(* Logix 5000 AddOnInstructionDefinition export HI6500_Faceplate_AOI; software revision 28.00 *)

ADD_ON_INSTRUCTION HI6500_Faceplate_AOI   (* revision 1.2 *)
VAR_IN_OUT
   Inp_hi6500 : _0102:Hardy6500Series_19FEEB66:I:0; {required}
   Out_hi6500 : _0102:Hardy6500Series_74A2D67F:O:0; {required}
END_VAR
VAR_OUTPUT
   hardy_6500_net_wt : REAL; {access Read Only}
   hardy_6500_counter : SINT; {access Read Only}
   hardy_6500_gross_wt : REAL; {access Read Only}
   hardy_6500_status : DINT; {access Read Only}
   hardy_6500_unit_status : INT; {access Read Only}
END_VAR
VAR_INPUT
   Set_FaceplateAnimation : DINT;
   rd_c2_cal : DINT;
   pm_4081 : DINT;
   pm_4082 : REAL;
   pm_4103 : DINT;
   pm_4101 : REAL;
   pm_4102 : REAL;
   rd_tra_cal : DINT;
   pm_4181 : REAL;
   pm_4182 : REAL;
   rd_fill : DINT;
   pm_2081 : DINT;
   pm_2082 : DINT;
   rd_ins : DINT;
   pm_2882 : DINT;
   pm_2883 : DINT;
   pm_2887 : REAL;
   pm_2888 : REAL;
   pm_2881 : DINT;
   rd_op2 : DINT;
   pm_2886 : REAL;
   pm_6182 : REAL;
   pm_6183 : REAL;
   pm_6303 : REAL;
   rd_az : DINT;
   pm_6301 : DINT;
   pm_6302 : REAL;
   pm_6381 : REAL;
   rd_iz : DINT;
   pm_6281 : DINT;
   pm_6282 : REAL;
   pm_6283 : REAL;
   pm_6284 : REAL;
   zero_cmd1 : DINT;
   tare_cmd : DINT;
   cal_low_cmd : DINT;
   cal_high_cmd : DINT;
   c2_cmd : DINT;
   control_bit : DINT;
   wr_cal_m_tol : DINT;
   fp_dis_md : DINT := 4;
   tare_zero_cmd : DINT;
   tare_zero_vl : DINT;
   wr_cell_sens : DINT;
   wr_wav_sav : DINT;
   wr_num_avg : DINT;
   wr_dec_pt : DINT;
   wr_grad : DINT;
   wr_mot_tol : DINT;
   wr_scal_cap : DINT;
   wr_unit : DINT;
   wr_ct_ena : DINT;
   pm_6104 : DINT;
   wr_un_wt : DINT;
   pm_6102 : REAL;
   wr_sm_size : DINT;
   pm_6103 : DINT;
   wr_dis_md : DINT;
   pm_8083 : DINT;
   wr_zr_tol : DINT;
   wr_tr_off : DINT;
   wr_tr_amt : DINT;
   wr_ref_wt : DINT;
   wr_gra_corr : DINT;
   wr_cal_lo_wt : DINT;
   wr_span_wt : DINT;
   wr_az_enable : DINT;
   wr_az_tol : DINT;
   wr_warm_time : DINT;
   wr_iz_enable : DINT;
   wr_plusiz_tol : DINT;
   wr_minusiz_tol : DINT;
   save_ins_pm : DINT;
   save_c2_pm : INT;
   save_op2_pm : INT;
   save_az_pm : INT;
   save_iz_pm : INT;
   save_tradcal_pm : INT;
   pm_6201 : REAL;
   Set_FaceplateHelpAnimation : DINT;
   wr_cal_m_tol_2 : INT;
   wr_nvm_cmd : DINT;
END_VAR
VAR_OUTPUT
   unit_flt : BOOL; {access Read Only}
   cal_status : DINT := 20; {access Read Only}
   status1 : DINT; {access Read Only}
END_VAR
VAR_INPUT
   save_fil_pm : INT;
END_VAR
VAR_OUTPUT
   instrument_status : DINT; {access Read Only}
END_VAR
VAR
   start_timer4 : BOOL; {access None}
   delay4 : TIMER := (PRE := 200); {access None}
   start_timer2 : BOOL; {access None}
   delay2 : TIMER := (PRE := 200); {access None}
   start_timer5 : BOOL; {access None}
   delay5 : TIMER := (PRE := 200); {access None}
   start_timer : BOOL; {access None}
   delay : TIMER := (PRE := 200); {access None}
   start_timer7 : BOOL; {access None}
   delay7 : TIMER := (PRE := 200); {access None}
   start_timer6 : BOOL; {access None}
   delay6 : TIMER := (PRE := 200); {access None}
   start_timer8 : BOOL; {access None}
   delay8 : TIMER := (PRE := 200); {access None}
   cmd_no : DINT; {access None}
   start_timer9 : BOOL; {access None}
   delay9 : TIMER := (PRE := 200); {access None}
   start_timer10 : BOOL; {access None}
   delay10 : TIMER := (PRE := 200); {access None}
   start_timer11 : BOOL; {access None}
   delay11 : TIMER := (PRE := 200); {access None}
   start_timer12 : BOOL; {access None}
   delay12 : TIMER := (PRE := 200); {access None}
   start_timer13 : BOOL; {access None}
   delay13 : TIMER := (PRE := 200); {access None}
   start_timer14 : BOOL; {access None}
   delay14 : TIMER := (PRE := 200); {access None}
   start_timer15 : BOOL; {access None}
   delay15 : TIMER := (PRE := 200); {access None}
   start_timer16 : BOOL; {access None}
   delay16 : TIMER := (PRE := 200); {access None}
   start_timer17 : BOOL; {access None}
   delay17 : TIMER := (PRE := 200); {access None}
   start_timer18 : BOOL; {access None}
   delay18 : TIMER := (PRE := 200); {access None}
   start_timer19 : BOOL; {access None}
   delay19 : TIMER := (PRE := 200); {access None}
   start_timer20 : BOOL; {access None}
   delay20 : TIMER := (PRE := 200); {access None}
   start_timer21 : BOOL; {access None}
   delay21 : TIMER := (PRE := 200); {access None}
   start_timer22 : BOOL; {access None}
   delay22 : TIMER := (PRE := 200); {access None}
   start_timer23 : BOOL; {access None}
   delay23 : TIMER := (PRE := 200); {access None}
   start_timer24 : BOOL; {access None}
   delay24 : TIMER := (PRE := 200); {access None}
   start_timer25 : BOOL; {access None}
   delay25 : TIMER := (PRE := 80); {access None}
   cmd_no_cal : DINT; {access None}
   start_timer26 : BOOL; {access None}
   delay26 : TIMER := (PRE := 200); {access None}
   start_timer27 : BOOL; {access None}
   delay27 : TIMER := (PRE := 200); {access None}
   start_timer28 : BOOL; {access None}
   delay28 : TIMER := (PRE := 200); {access None}
   start_timer29 : BOOL; {access None}
   delay29 : TIMER := (PRE := 200); {access None}
   start_timer30 : BOOL; {access None}
   delay30 : TIMER := (PRE := 200); {access None}
   wr_cell_sens2 : INT; {access None}
   start_timer31 : BOOL; {access None}
   delay31 : TIMER := (PRE := 200); {access None}
   start_timer32 : BOOL; {access None}
   delay32 : TIMER := (PRE := 200); {access None}
   start_timer33 : BOOL; {access None}
   delay33 : TIMER := (PRE := 200); {access None}
   temp : BOOL; {access None}
   temp3 : BOOL; {access None}
   timer35 : TIMER := (PRE := 4000); {access None}
   temp2 : BOOL; {access None}
   temp4 : BOOL; {access None}
   temp5 : BOOL; {access None}
   temp6 : BOOL; {access None}
   temp7 : BOOL; {access None}
   temp8 : BOOL; {access None}
   temp9 : BOOL; {access None}
   temp10 : BOOL; {access None}
   temp11 : BOOL; {access None}
   temp12 : BOOL; {access None}
   temp13 : BOOL; {access None}
   temp14 : BOOL; {access None}
   temp15 : BOOL; {access None}
   temp16 : BOOL; {access None}
   temp17 : BOOL; {access None}
   temp18 : BOOL; {access None}
   temp19 : BOOL; {access None}
   temp20 : BOOL; {access None}
   temp21 : BOOL; {access None}
   temp22 : BOOL; {access None}
   temp23 : BOOL; {access None}
   temp24 : BOOL; {access None}
   temp25 : BOOL; {access None}
   temp26 : BOOL; {access None}
   temp27 : BOOL; {access None}
   temp28 : BOOL; {access None}
   temp29 : BOOL; {access None}
   temp100 : BOOL; {access None}
   blk : BOOL; {access None}
   timer38 : TIMER := (PRE := 2000); {access None}
   timer39 : TIMER := (PRE := 2000); {access None}
   temp42 : BOOL; {access None}
   temp41 : BOOL; {access None}
END_VAR

ROUTINE Logic   (* ladder *)
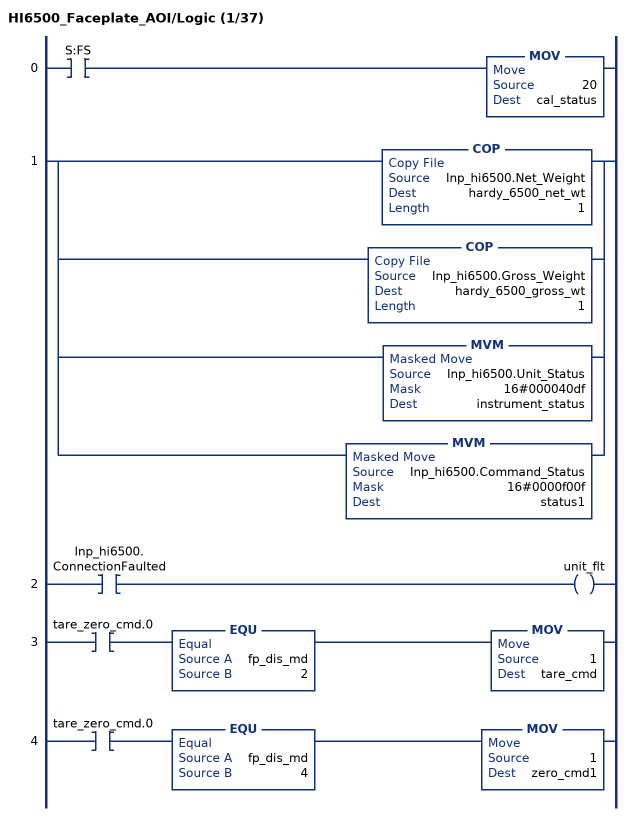
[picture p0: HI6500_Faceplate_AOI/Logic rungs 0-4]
   0: XIC(S:FS)MOV(20,cal_status);
   1: [COP(Inp_hi6500.Net_Weight,hardy_6500_net_wt,1) ,COP(Inp_hi6500.Gross_Weight,hardy_6500_gross_wt,1) ,MVM(Inp_hi6500.Unit_Status,16#000040df,instrument_status) ,MVM(Inp_hi6500.Command_Status,16#0000f00f,status1) ];
   2: XIC(Inp_hi6500.ConnectionFaulted)OTE(unit_flt);
   3: XIC(tare_zero_cmd.0)EQU(fp_dis_md,2)MOV(1,tare_cmd);
   4: XIC(tare_zero_cmd.0)EQU(fp_dis_md,4)MOV(1,zero_cmd1);
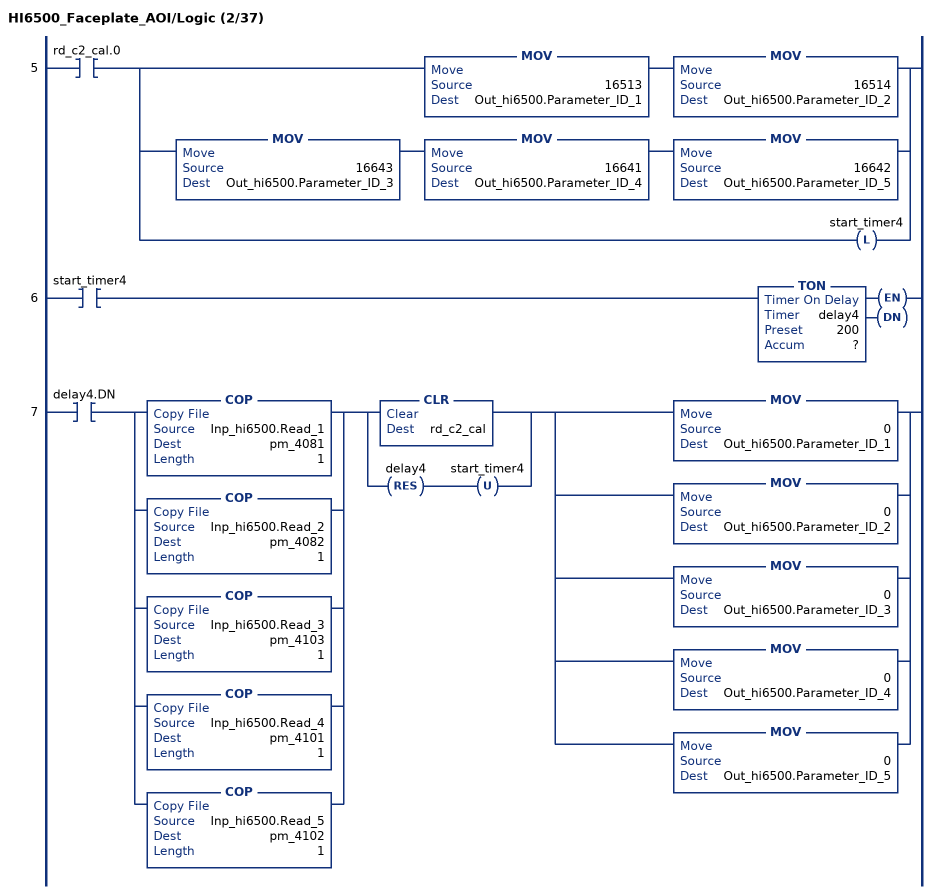
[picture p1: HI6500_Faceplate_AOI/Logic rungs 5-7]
   5: XIC(rd_c2_cal.0)[MOV(16513,Out_hi6500.Parameter_ID_1) MOV(16514,Out_hi6500.Parameter_ID_2) ,MOV(16643,Out_hi6500.Parameter_ID_3) MOV(16641,Out_hi6500.Parameter_ID_4) MOV(16642,Out_hi6500.Parameter_ID_5) ,OTL(start_timer4) ];
   6: XIC(start_timer4)TON(delay4,?,?);
   7: XIC(delay4.DN)[COP(Inp_hi6500.Read_1,pm_4081,1) ,COP(Inp_hi6500.Read_2,pm_4082,1) ,COP(Inp_hi6500.Read_3,pm_4103,1) ,COP(Inp_hi6500.Read_4,pm_4101,1) ,COP(Inp_hi6500.Read_5,pm_4102,1) ][CLR(rd_c2_cal) ,RES(delay4) OTU(start_timer4) ][MOV(0,Out_hi6500.Parameter_ID_1) ,MOV(0,Out_hi6500.Parameter_ID_2) ,MOV(0,Out_hi6500.Parameter_ID_3) ,MOV(0,Out_hi6500.Parameter_ID_4) ,MOV(0,Out_hi6500.Parameter_ID_5) ];
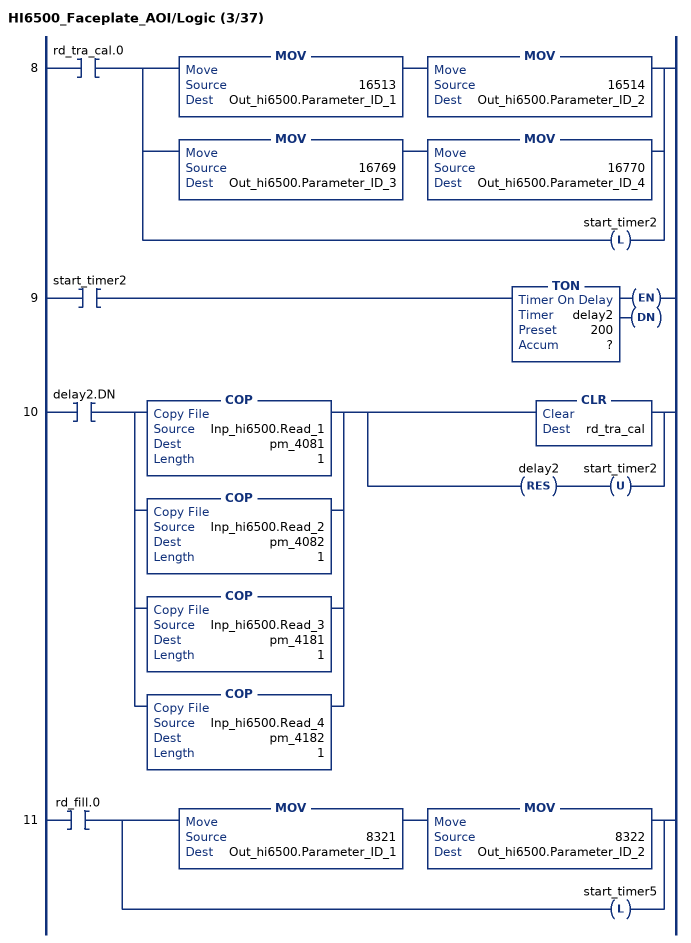
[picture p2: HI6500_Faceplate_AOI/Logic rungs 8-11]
   8: XIC(rd_tra_cal.0)[MOV(16513,Out_hi6500.Parameter_ID_1) MOV(16514,Out_hi6500.Parameter_ID_2) ,MOV(16769,Out_hi6500.Parameter_ID_3) MOV(16770,Out_hi6500.Parameter_ID_4) ,OTL(start_timer2) ];
   9: XIC(start_timer2)TON(delay2,?,?);
   10: XIC(delay2.DN)[COP(Inp_hi6500.Read_1,pm_4081,1) ,COP(Inp_hi6500.Read_2,pm_4082,1) ,COP(Inp_hi6500.Read_3,pm_4181,1) ,COP(Inp_hi6500.Read_4,pm_4182,1) ][CLR(rd_tra_cal) ,RES(delay2) OTU(start_timer2) ];
   11: XIC(rd_fill.0)[MOV(8321,Out_hi6500.Parameter_ID_1) MOV(8322,Out_hi6500.Parameter_ID_2) ,OTL(start_timer5) ];
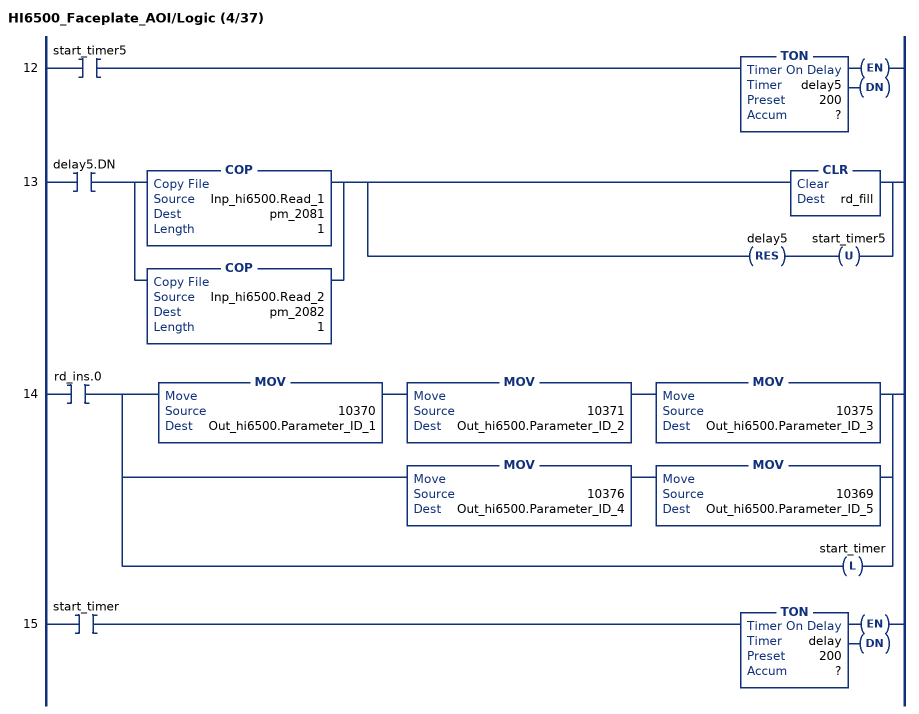
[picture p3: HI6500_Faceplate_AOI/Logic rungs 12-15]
   12: XIC(start_timer5)TON(delay5,?,?);
   13: XIC(delay5.DN)[COP(Inp_hi6500.Read_1,pm_2081,1) ,COP(Inp_hi6500.Read_2,pm_2082,1) ][CLR(rd_fill) ,RES(delay5) OTU(start_timer5) ];
   14: XIC(rd_ins.0)[MOV(10370,Out_hi6500.Parameter_ID_1) MOV(10371,Out_hi6500.Parameter_ID_2) MOV(10375,Out_hi6500.Parameter_ID_3) ,MOV(10376,Out_hi6500.Parameter_ID_4) MOV(10369,Out_hi6500.Parameter_ID_5) ,OTL(start_timer) ];
   15: XIC(start_timer)TON(delay,?,?);
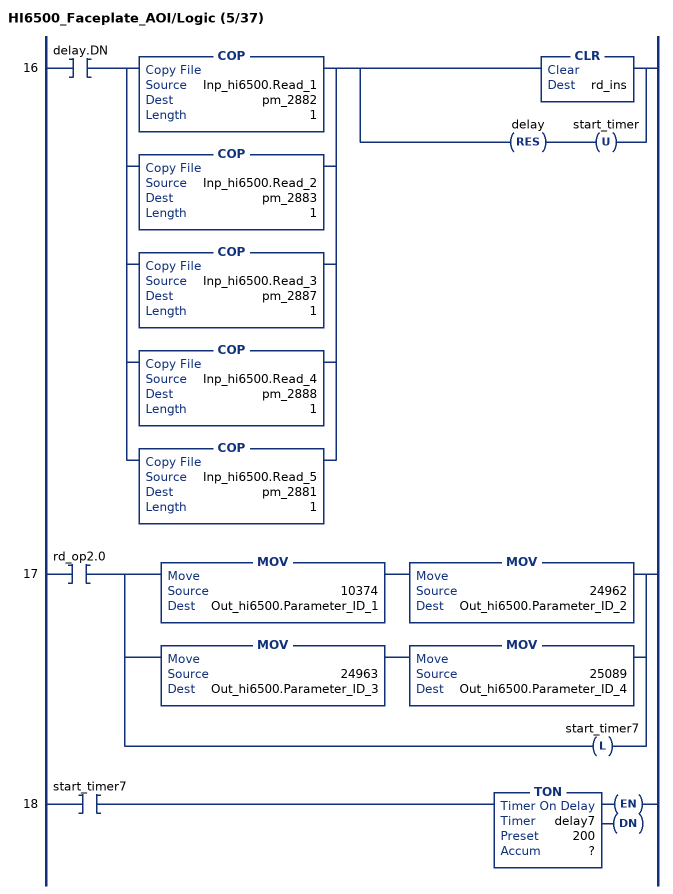
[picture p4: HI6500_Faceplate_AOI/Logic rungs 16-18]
   16: XIC(delay.DN)[COP(Inp_hi6500.Read_1,pm_2882,1) ,COP(Inp_hi6500.Read_2,pm_2883,1) ,COP(Inp_hi6500.Read_3,pm_2887,1) ,COP(Inp_hi6500.Read_4,pm_2888,1) ,COP(Inp_hi6500.Read_5,pm_2881,1) ][CLR(rd_ins) ,RES(delay) OTU(start_timer) ];
   17: XIC(rd_op2.0)[MOV(10374,Out_hi6500.Parameter_ID_1) MOV(24962,Out_hi6500.Parameter_ID_2) ,MOV(24963,Out_hi6500.Parameter_ID_3) MOV(25089,Out_hi6500.Parameter_ID_4) ,OTL(start_timer7) ];
   18: XIC(start_timer7)TON(delay7,?,?);
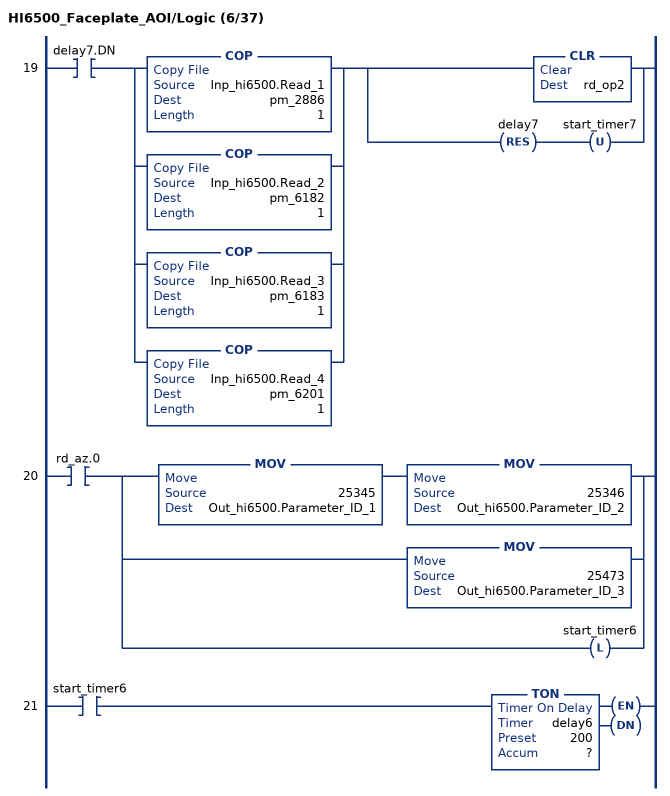
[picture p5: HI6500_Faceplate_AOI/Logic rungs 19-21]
   19: XIC(delay7.DN)[COP(Inp_hi6500.Read_1,pm_2886,1) ,COP(Inp_hi6500.Read_2,pm_6182,1) ,COP(Inp_hi6500.Read_3,pm_6183,1) ,COP(Inp_hi6500.Read_4,pm_6201,1) ][CLR(rd_op2) ,RES(delay7) OTU(start_timer7) ];
   20: XIC(rd_az.0)[MOV(25345,Out_hi6500.Parameter_ID_1) MOV(25346,Out_hi6500.Parameter_ID_2) ,MOV(25473,Out_hi6500.Parameter_ID_3) ,OTL(start_timer6) ];
   21: XIC(start_timer6)TON(delay6,?,?);
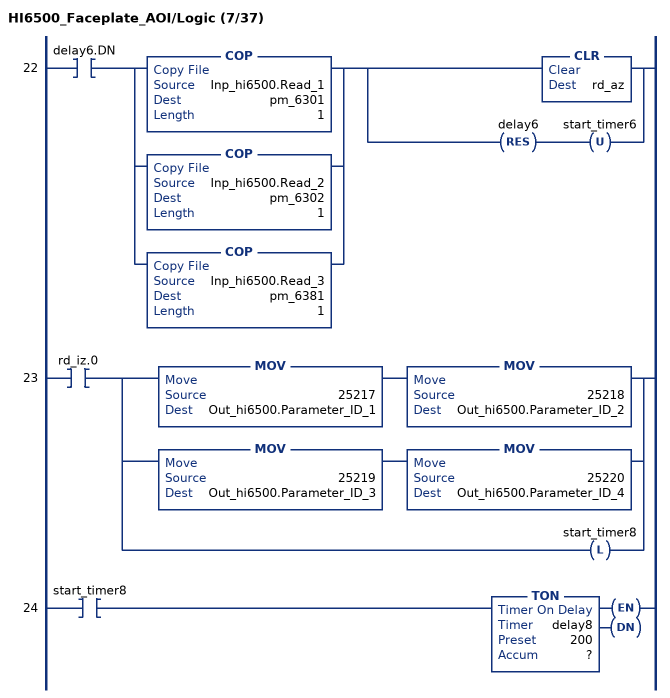
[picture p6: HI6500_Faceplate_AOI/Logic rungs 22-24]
   22: XIC(delay6.DN)[COP(Inp_hi6500.Read_1,pm_6301,1) ,COP(Inp_hi6500.Read_2,pm_6302,1) ,COP(Inp_hi6500.Read_3,pm_6381,1) ][CLR(rd_az) ,RES(delay6) OTU(start_timer6) ];
   23: XIC(rd_iz.0)[MOV(25217,Out_hi6500.Parameter_ID_1) MOV(25218,Out_hi6500.Parameter_ID_2) ,MOV(25219,Out_hi6500.Parameter_ID_3) MOV(25220,Out_hi6500.Parameter_ID_4) ,OTL(start_timer8) ];
   24: XIC(start_timer8)TON(delay8,?,?);
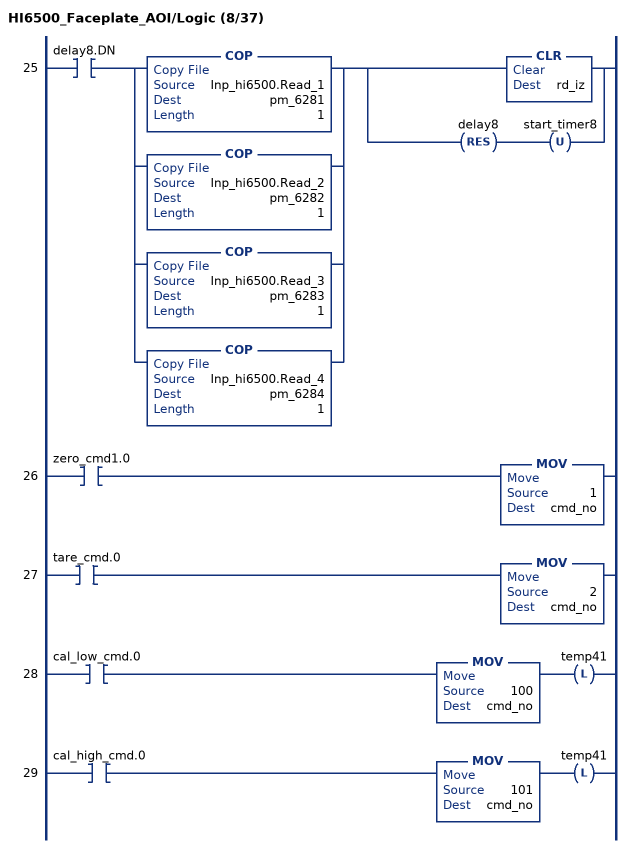
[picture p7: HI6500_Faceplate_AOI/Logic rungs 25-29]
   25: XIC(delay8.DN)[COP(Inp_hi6500.Read_1,pm_6281,1) ,COP(Inp_hi6500.Read_2,pm_6282,1) ,COP(Inp_hi6500.Read_3,pm_6283,1) ,COP(Inp_hi6500.Read_4,pm_6284,1) ][CLR(rd_iz) ,RES(delay8) OTU(start_timer8) ];
   26: XIC(zero_cmd1.0)MOV(1,cmd_no);
   27: XIC(tare_cmd.0)MOV(2,cmd_no);
   28: XIC(cal_low_cmd.0)MOV(100,cmd_no)OTL(temp41);
   29: XIC(cal_high_cmd.0)MOV(101,cmd_no)OTL(temp41);
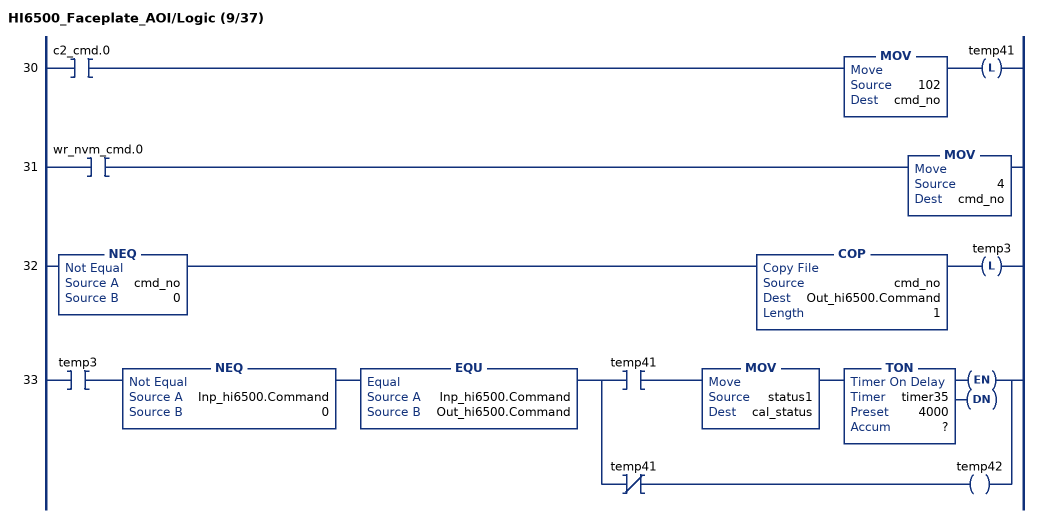
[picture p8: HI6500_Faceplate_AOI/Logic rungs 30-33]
   30: XIC(c2_cmd.0)MOV(102,cmd_no)OTL(temp41);
   31: XIC(wr_nvm_cmd.0)MOV(4,cmd_no);
   32: NEQ(cmd_no,0)COP(cmd_no,Out_hi6500.Command,1)OTL(temp3);
   33: XIC(temp3)NEQ(Inp_hi6500.Command,0)EQU(Inp_hi6500.Command,Out_hi6500.Command)[XIC(temp41) MOV(status1,cal_status) TON(timer35,?,?) ,XIO(temp41) OTE(temp42) ];
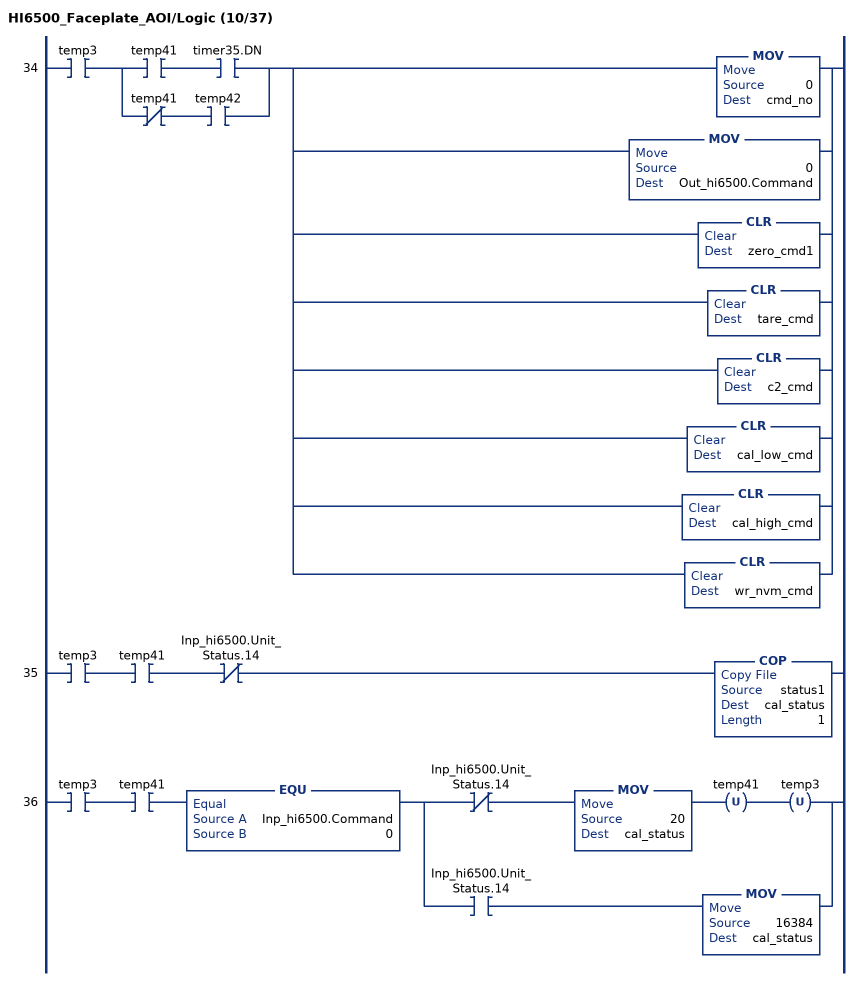
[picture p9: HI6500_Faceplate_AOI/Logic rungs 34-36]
   34: XIC(temp3)[XIC(temp41) XIC(timer35.DN) ,XIO(temp41) XIC(temp42) ][MOV(0,cmd_no) ,MOV(0,Out_hi6500.Command) ,CLR(zero_cmd1) ,CLR(tare_cmd) ,CLR(c2_cmd) ,CLR(cal_low_cmd) ,CLR(cal_high_cmd) ,CLR(wr_nvm_cmd) ];
   35: XIC(temp3)XIC(temp41)XIO(Inp_hi6500.Unit_Status.14)COP(status1,cal_status,1);
   36: XIC(temp3)XIC(temp41)EQU(Inp_hi6500.Command,0)[XIO(Inp_hi6500.Unit_Status.14) MOV(20,cal_status) OTU(temp41) OTU(temp3) ,XIC(Inp_hi6500.Unit_Status.14) MOV(16384,cal_status) ];
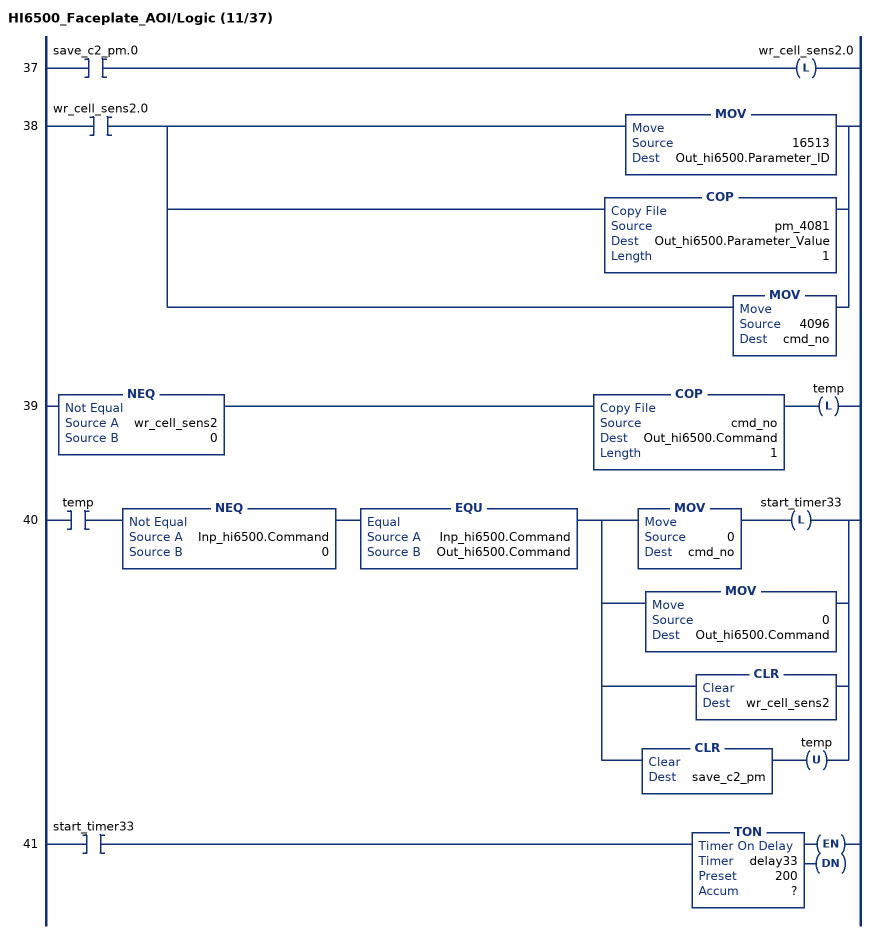
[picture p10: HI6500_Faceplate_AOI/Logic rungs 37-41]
   37: XIC(save_c2_pm.0)OTL(wr_cell_sens2.0);
   38: XIC(wr_cell_sens2.0)[MOV(16513,Out_hi6500.Parameter_ID) ,COP(pm_4081,Out_hi6500.Parameter_Value,1) ,MOV(4096,cmd_no) ];
   39: NEQ(wr_cell_sens2,0)COP(cmd_no,Out_hi6500.Command,1)OTL(temp);
   40: XIC(temp)NEQ(Inp_hi6500.Command,0)EQU(Inp_hi6500.Command,Out_hi6500.Command)[MOV(0,cmd_no) OTL(start_timer33) ,MOV(0,Out_hi6500.Command) ,CLR(wr_cell_sens2) ,CLR(save_c2_pm) OTU(temp) ];
   41: XIC(start_timer33)TON(delay33,?,?);
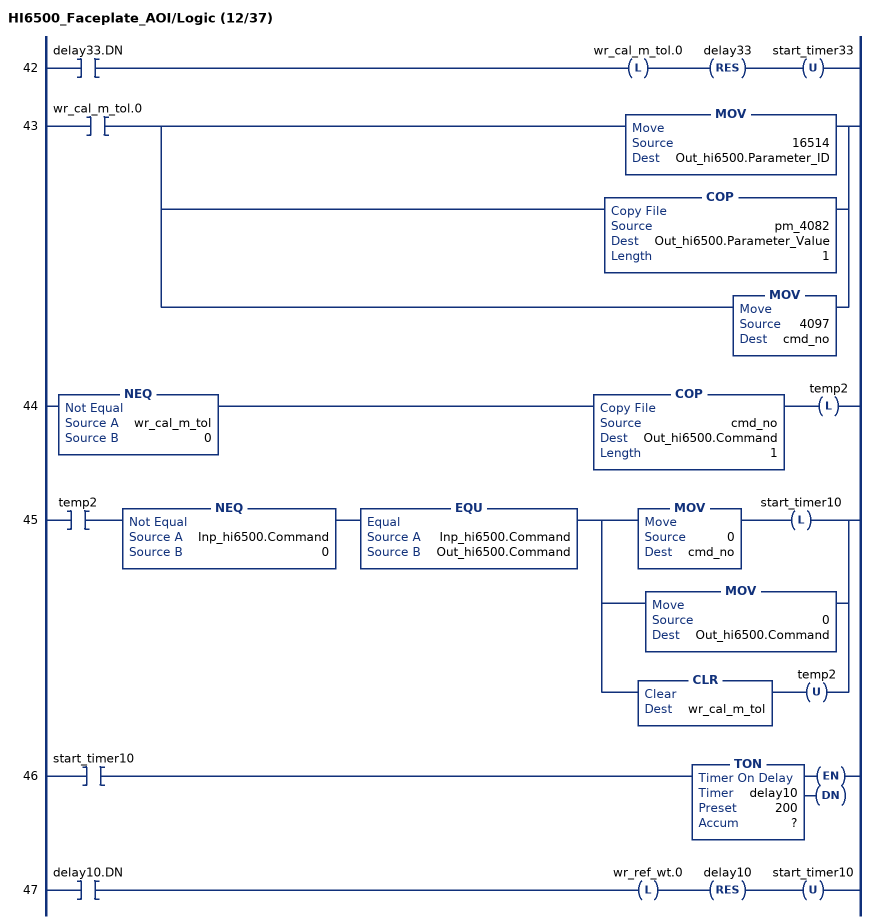
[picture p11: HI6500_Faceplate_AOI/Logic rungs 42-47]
   42: XIC(delay33.DN)OTL(wr_cal_m_tol.0)RES(delay33)OTU(start_timer33);
   43: XIC(wr_cal_m_tol.0)[MOV(16514,Out_hi6500.Parameter_ID) ,COP(pm_4082,Out_hi6500.Parameter_Value,1) ,MOV(4097,cmd_no) ];
   44: NEQ(wr_cal_m_tol,0)COP(cmd_no,Out_hi6500.Command,1)OTL(temp2);
   45: XIC(temp2)NEQ(Inp_hi6500.Command,0)EQU(Inp_hi6500.Command,Out_hi6500.Command)[MOV(0,cmd_no) OTL(start_timer10) ,MOV(0,Out_hi6500.Command) ,CLR(wr_cal_m_tol) OTU(temp2) ];
   46: XIC(start_timer10)TON(delay10,?,?);
   47: XIC(delay10.DN)OTL(wr_ref_wt.0)RES(delay10)OTU(start_timer10);
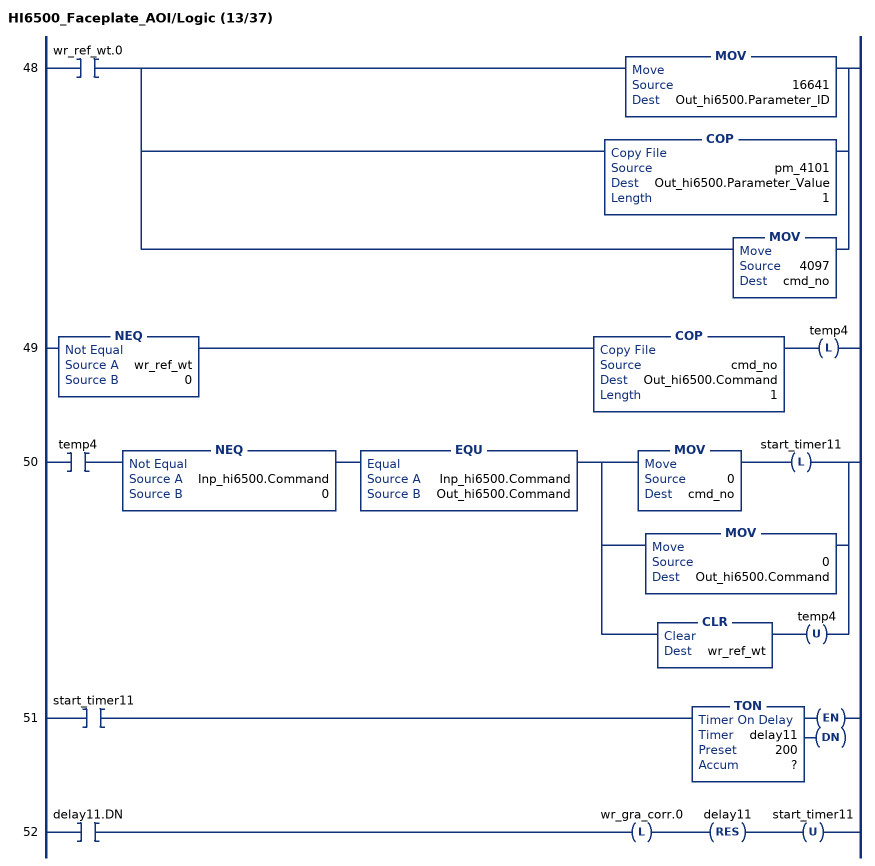
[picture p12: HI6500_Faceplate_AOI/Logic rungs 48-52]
   48: XIC(wr_ref_wt.0)[MOV(16641,Out_hi6500.Parameter_ID) ,COP(pm_4101,Out_hi6500.Parameter_Value,1) ,MOV(4097,cmd_no) ];
   49: NEQ(wr_ref_wt,0)COP(cmd_no,Out_hi6500.Command,1)OTL(temp4);
   50: XIC(temp4)NEQ(Inp_hi6500.Command,0)EQU(Inp_hi6500.Command,Out_hi6500.Command)[MOV(0,cmd_no) OTL(start_timer11) ,MOV(0,Out_hi6500.Command) ,CLR(wr_ref_wt) OTU(temp4) ];
   51: XIC(start_timer11)TON(delay11,?,?);
   52: XIC(delay11.DN)OTL(wr_gra_corr.0)RES(delay11)OTU(start_timer11);
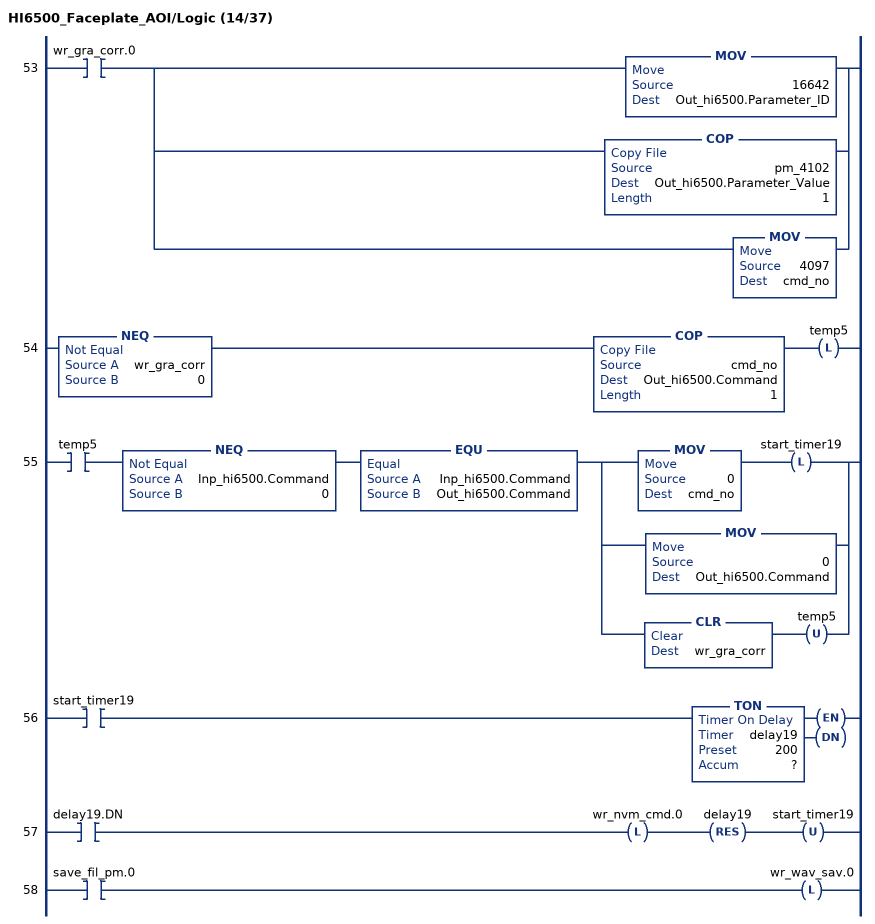
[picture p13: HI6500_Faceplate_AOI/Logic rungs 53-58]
   53: XIC(wr_gra_corr.0)[MOV(16642,Out_hi6500.Parameter_ID) ,COP(pm_4102,Out_hi6500.Parameter_Value,1) ,MOV(4097,cmd_no) ];
   54: NEQ(wr_gra_corr,0)COP(cmd_no,Out_hi6500.Command,1)OTL(temp5);
   55: XIC(temp5)NEQ(Inp_hi6500.Command,0)EQU(Inp_hi6500.Command,Out_hi6500.Command)[MOV(0,cmd_no) OTL(start_timer19) ,MOV(0,Out_hi6500.Command) ,CLR(wr_gra_corr) OTU(temp5) ];
   56: XIC(start_timer19)TON(delay19,?,?);
   57: XIC(delay19.DN)OTL(wr_nvm_cmd.0)RES(delay19)OTU(start_timer19);
   58: XIC(save_fil_pm.0)OTL(wr_wav_sav.0);
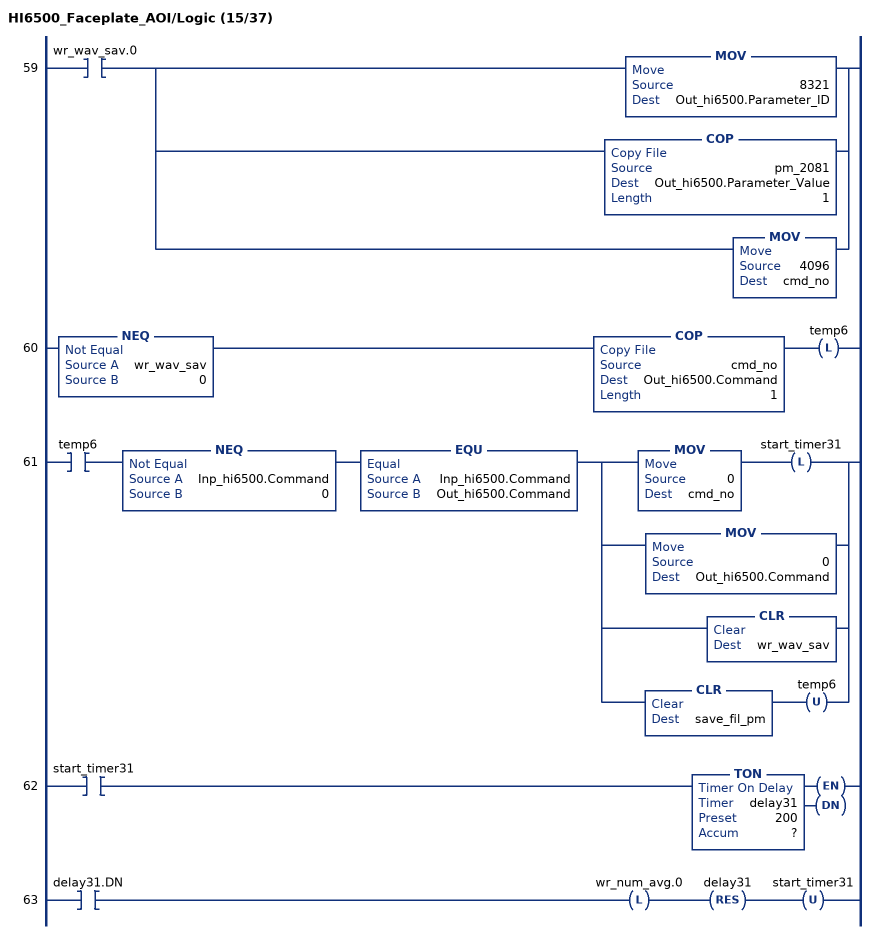
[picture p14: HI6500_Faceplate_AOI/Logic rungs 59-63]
   59: XIC(wr_wav_sav.0)[MOV(8321,Out_hi6500.Parameter_ID) ,COP(pm_2081,Out_hi6500.Parameter_Value,1) ,MOV(4096,cmd_no) ];
   60: NEQ(wr_wav_sav,0)COP(cmd_no,Out_hi6500.Command,1)OTL(temp6);
   61: XIC(temp6)NEQ(Inp_hi6500.Command,0)EQU(Inp_hi6500.Command,Out_hi6500.Command)[MOV(0,cmd_no) OTL(start_timer31) ,MOV(0,Out_hi6500.Command) ,CLR(wr_wav_sav) ,CLR(save_fil_pm) OTU(temp6) ];
   62: XIC(start_timer31)TON(delay31,?,?);
   63: XIC(delay31.DN)OTL(wr_num_avg.0)RES(delay31)OTU(start_timer31);
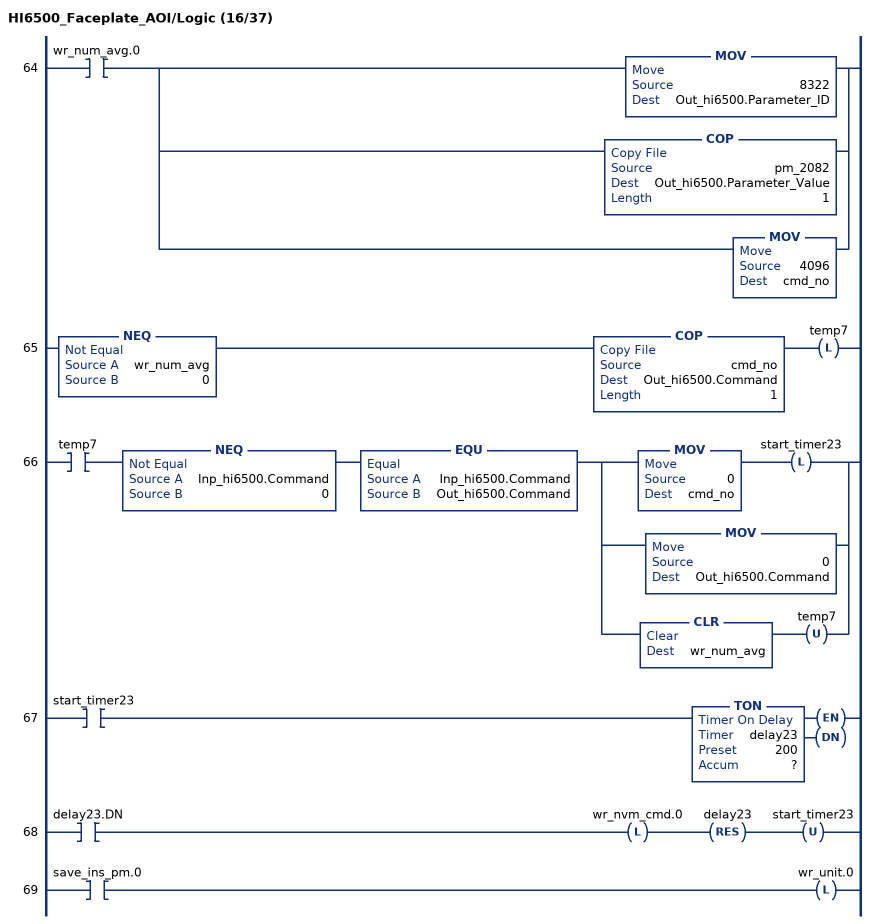
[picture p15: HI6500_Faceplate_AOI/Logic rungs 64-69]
   64: XIC(wr_num_avg.0)[MOV(8322,Out_hi6500.Parameter_ID) ,COP(pm_2082,Out_hi6500.Parameter_Value,1) ,MOV(4096,cmd_no) ];
   65: NEQ(wr_num_avg,0)COP(cmd_no,Out_hi6500.Command,1)OTL(temp7);
   66: XIC(temp7)NEQ(Inp_hi6500.Command,0)EQU(Inp_hi6500.Command,Out_hi6500.Command)[MOV(0,cmd_no) OTL(start_timer23) ,MOV(0,Out_hi6500.Command) ,CLR(wr_num_avg) OTU(temp7) ];
   67: XIC(start_timer23)TON(delay23,?,?);
   68: XIC(delay23.DN)OTL(wr_nvm_cmd.0)RES(delay23)OTU(start_timer23);
   69: XIC(save_ins_pm.0)OTL(wr_unit.0);
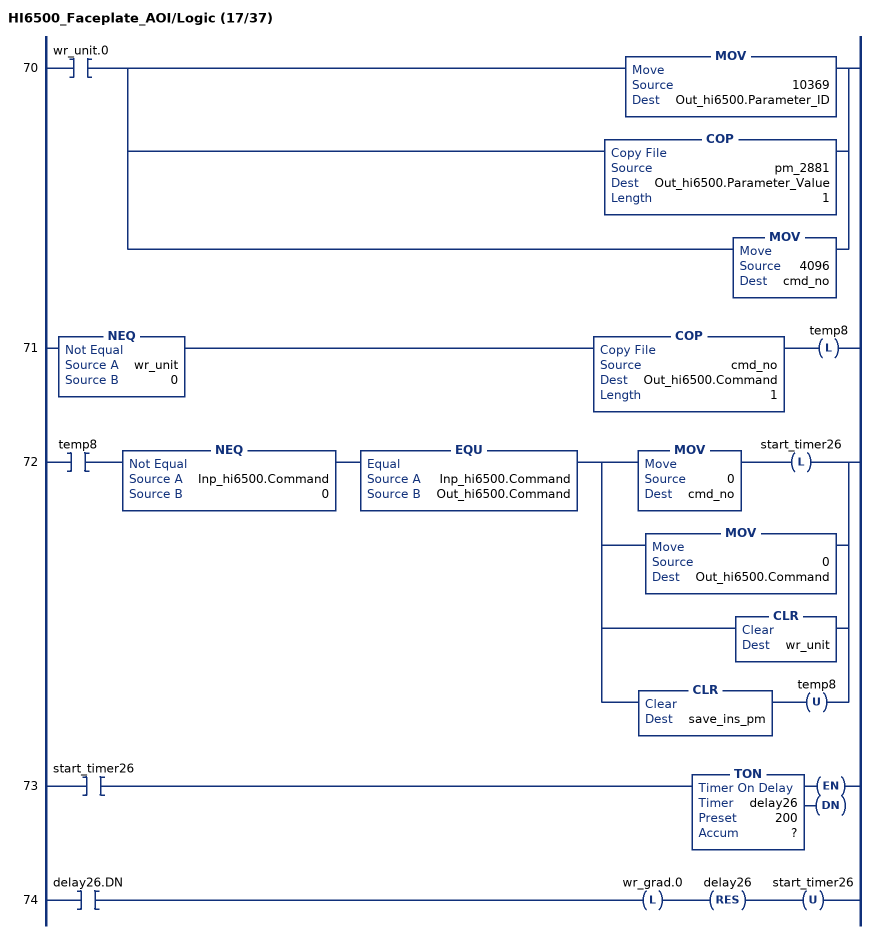
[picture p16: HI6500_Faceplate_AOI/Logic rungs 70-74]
   70: XIC(wr_unit.0)[MOV(10369,Out_hi6500.Parameter_ID) ,COP(pm_2881,Out_hi6500.Parameter_Value,1) ,MOV(4096,cmd_no) ];
   71: NEQ(wr_unit,0)COP(cmd_no,Out_hi6500.Command,1)OTL(temp8);
   72: XIC(temp8)NEQ(Inp_hi6500.Command,0)EQU(Inp_hi6500.Command,Out_hi6500.Command)[MOV(0,cmd_no) OTL(start_timer26) ,MOV(0,Out_hi6500.Command) ,CLR(wr_unit) ,CLR(save_ins_pm) OTU(temp8) ];
   73: XIC(start_timer26)TON(delay26,?,?);
   74: XIC(delay26.DN)OTL(wr_grad.0)RES(delay26)OTU(start_timer26);
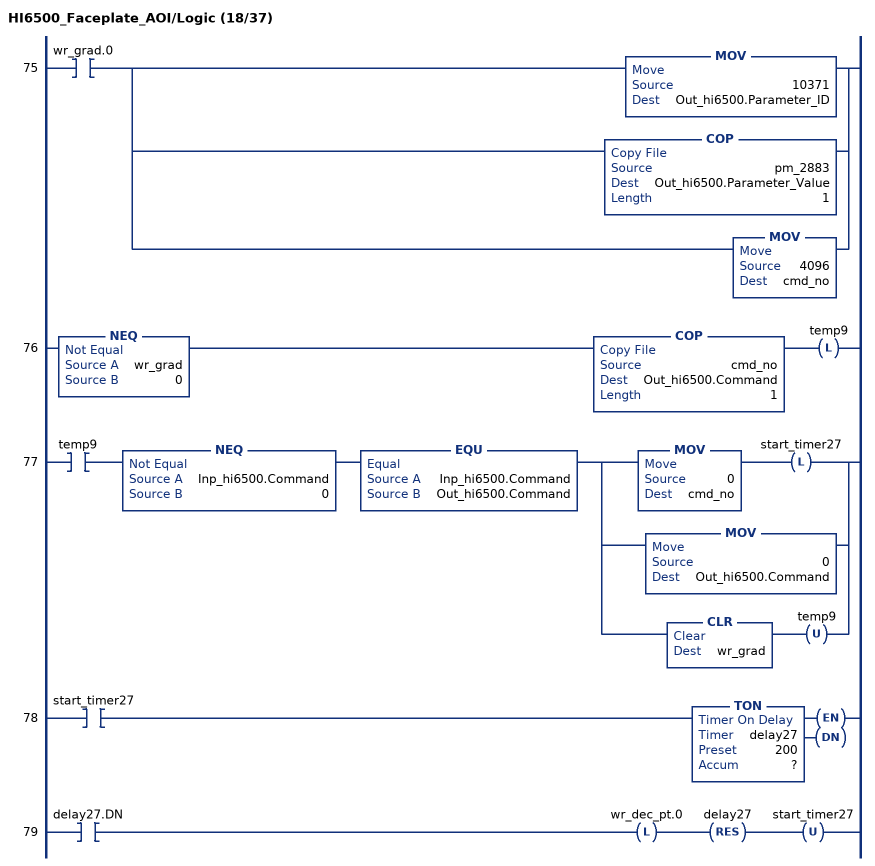
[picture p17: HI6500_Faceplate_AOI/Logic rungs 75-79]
   75: XIC(wr_grad.0)[MOV(10371,Out_hi6500.Parameter_ID) ,COP(pm_2883,Out_hi6500.Parameter_Value,1) ,MOV(4096,cmd_no) ];
   76: NEQ(wr_grad,0)COP(cmd_no,Out_hi6500.Command,1)OTL(temp9);
   77: XIC(temp9)NEQ(Inp_hi6500.Command,0)EQU(Inp_hi6500.Command,Out_hi6500.Command)[MOV(0,cmd_no) OTL(start_timer27) ,MOV(0,Out_hi6500.Command) ,CLR(wr_grad) OTU(temp9) ];
   78: XIC(start_timer27)TON(delay27,?,?);
   79: XIC(delay27.DN)OTL(wr_dec_pt.0)RES(delay27)OTU(start_timer27);
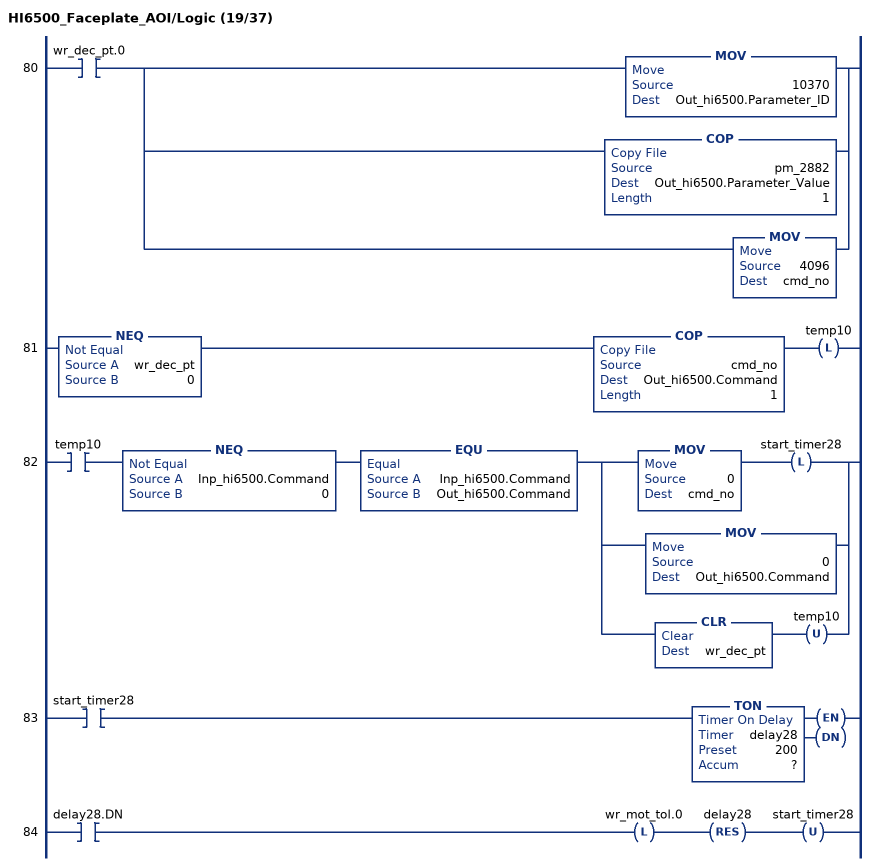
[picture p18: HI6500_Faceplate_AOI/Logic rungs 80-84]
   80: XIC(wr_dec_pt.0)[MOV(10370,Out_hi6500.Parameter_ID) ,COP(pm_2882,Out_hi6500.Parameter_Value,1) ,MOV(4096,cmd_no) ];
   81: NEQ(wr_dec_pt,0)COP(cmd_no,Out_hi6500.Command,1)OTL(temp10);
   82: XIC(temp10)NEQ(Inp_hi6500.Command,0)EQU(Inp_hi6500.Command,Out_hi6500.Command)[MOV(0,cmd_no) OTL(start_timer28) ,MOV(0,Out_hi6500.Command) ,CLR(wr_dec_pt) OTU(temp10) ];
   83: XIC(start_timer28)TON(delay28,?,?);
   84: XIC(delay28.DN)OTL(wr_mot_tol.0)RES(delay28)OTU(start_timer28);
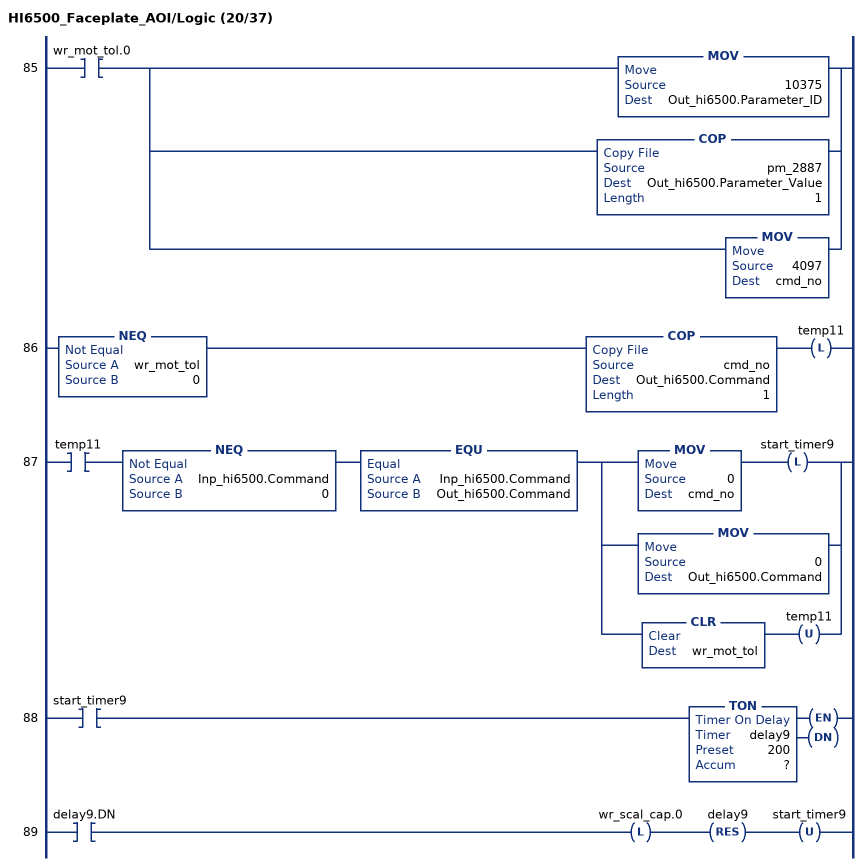
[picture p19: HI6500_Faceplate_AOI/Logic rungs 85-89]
   85: XIC(wr_mot_tol.0)[MOV(10375,Out_hi6500.Parameter_ID) ,COP(pm_2887,Out_hi6500.Parameter_Value,1) ,MOV(4097,cmd_no) ];
   86: NEQ(wr_mot_tol,0)COP(cmd_no,Out_hi6500.Command,1)OTL(temp11);
   87: XIC(temp11)NEQ(Inp_hi6500.Command,0)EQU(Inp_hi6500.Command,Out_hi6500.Command)[MOV(0,cmd_no) OTL(start_timer9) ,MOV(0,Out_hi6500.Command) ,CLR(wr_mot_tol) OTU(temp11) ];
   88: XIC(start_timer9)TON(delay9,?,?);
   89: XIC(delay9.DN)OTL(wr_scal_cap.0)RES(delay9)OTU(start_timer9);
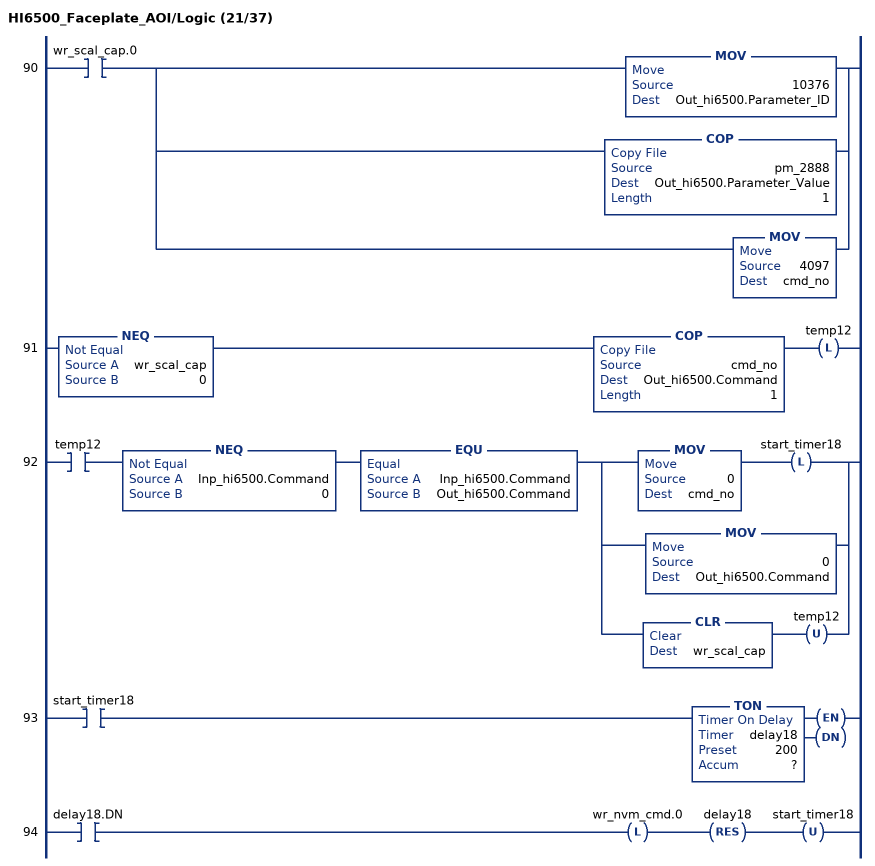
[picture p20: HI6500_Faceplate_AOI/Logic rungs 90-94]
   90: XIC(wr_scal_cap.0)[MOV(10376,Out_hi6500.Parameter_ID) ,COP(pm_2888,Out_hi6500.Parameter_Value,1) ,MOV(4097,cmd_no) ];
   91: NEQ(wr_scal_cap,0)COP(cmd_no,Out_hi6500.Command,1)OTL(temp12);
   92: XIC(temp12)NEQ(Inp_hi6500.Command,0)EQU(Inp_hi6500.Command,Out_hi6500.Command)[MOV(0,cmd_no) OTL(start_timer18) ,MOV(0,Out_hi6500.Command) ,CLR(wr_scal_cap) OTU(temp12) ];
   93: XIC(start_timer18)TON(delay18,?,?);
   94: XIC(delay18.DN)OTL(wr_nvm_cmd.0)RES(delay18)OTU(start_timer18);
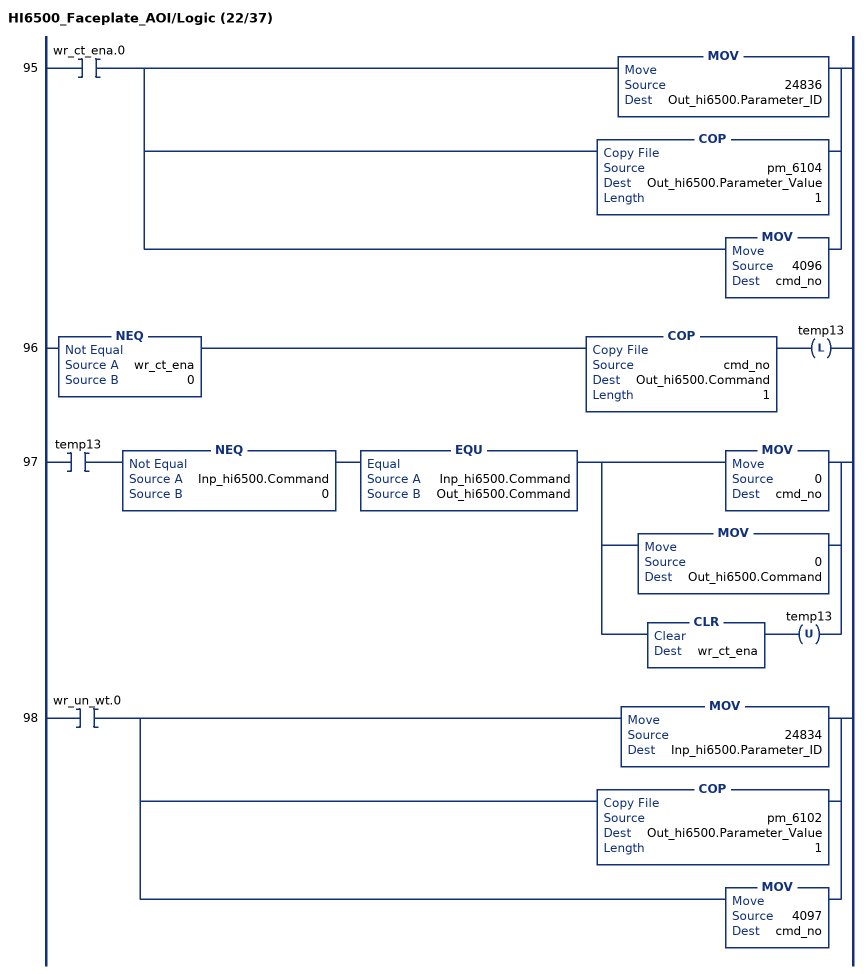
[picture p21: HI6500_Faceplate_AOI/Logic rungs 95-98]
   95: XIC(wr_ct_ena.0)[MOV(24836,Out_hi6500.Parameter_ID) ,COP(pm_6104,Out_hi6500.Parameter_Value,1) ,MOV(4096,cmd_no) ];
   96: NEQ(wr_ct_ena,0)COP(cmd_no,Out_hi6500.Command,1)OTL(temp13);
   97: XIC(temp13)NEQ(Inp_hi6500.Command,0)EQU(Inp_hi6500.Command,Out_hi6500.Command)[MOV(0,cmd_no) ,MOV(0,Out_hi6500.Command) ,CLR(wr_ct_ena) OTU(temp13) ];
   98: XIC(wr_un_wt.0)[MOV(24834,Inp_hi6500.Parameter_ID) ,COP(pm_6102,Out_hi6500.Parameter_Value,1) ,MOV(4097,cmd_no) ];
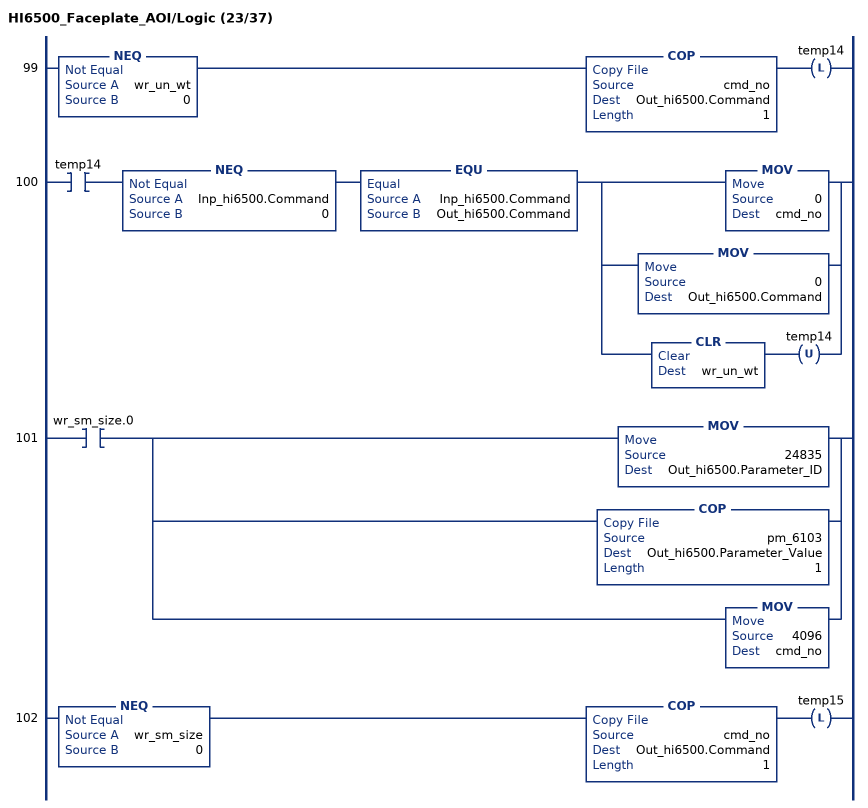
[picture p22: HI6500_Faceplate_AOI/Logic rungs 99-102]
   99: NEQ(wr_un_wt,0)COP(cmd_no,Out_hi6500.Command,1)OTL(temp14);
   100: XIC(temp14)NEQ(Inp_hi6500.Command,0)EQU(Inp_hi6500.Command,Out_hi6500.Command)[MOV(0,cmd_no) ,MOV(0,Out_hi6500.Command) ,CLR(wr_un_wt) OTU(temp14) ];
   101: XIC(wr_sm_size.0)[MOV(24835,Out_hi6500.Parameter_ID) ,COP(pm_6103,Out_hi6500.Parameter_Value,1) ,MOV(4096,cmd_no) ];
   102: NEQ(wr_sm_size,0)COP(cmd_no,Out_hi6500.Command,1)OTL(temp15);
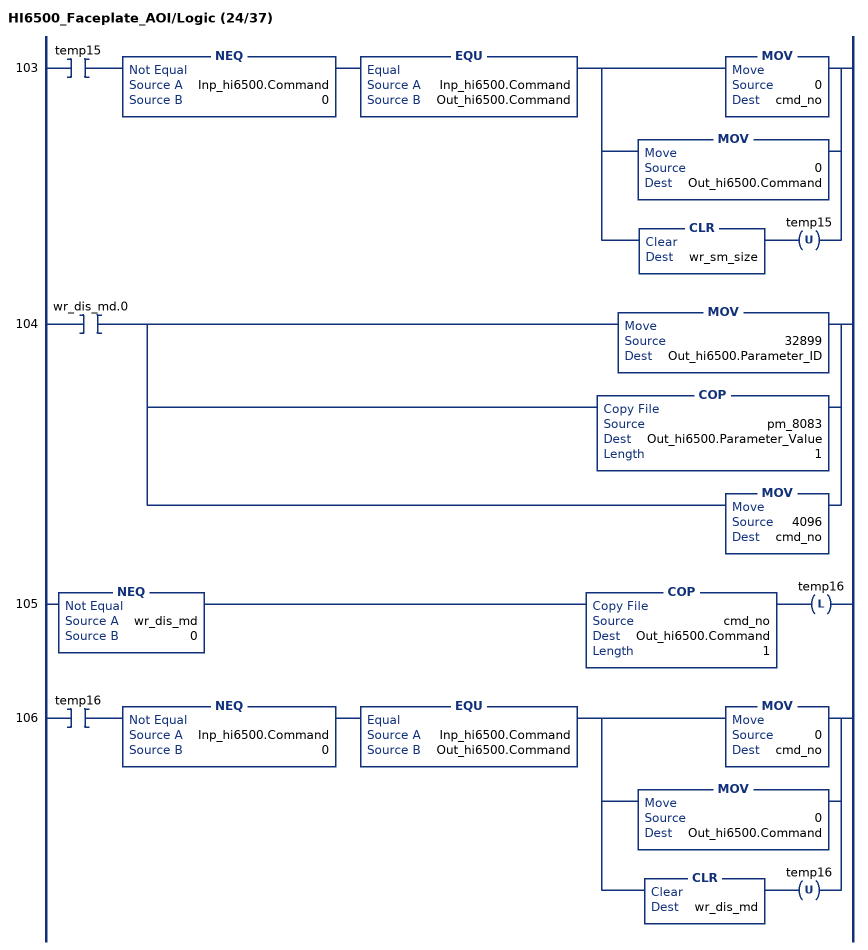
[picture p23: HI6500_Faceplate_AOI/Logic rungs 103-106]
   103: XIC(temp15)NEQ(Inp_hi6500.Command,0)EQU(Inp_hi6500.Command,Out_hi6500.Command)[MOV(0,cmd_no) ,MOV(0,Out_hi6500.Command) ,CLR(wr_sm_size) OTU(temp15) ];
   104: XIC(wr_dis_md.0)[MOV(32899,Out_hi6500.Parameter_ID) ,COP(pm_8083,Out_hi6500.Parameter_Value,1) ,MOV(4096,cmd_no) ];
   105: NEQ(wr_dis_md,0)COP(cmd_no,Out_hi6500.Command,1)OTL(temp16);
   106: XIC(temp16)NEQ(Inp_hi6500.Command,0)EQU(Inp_hi6500.Command,Out_hi6500.Command)[MOV(0,cmd_no) ,MOV(0,Out_hi6500.Command) ,CLR(wr_dis_md) OTU(temp16) ];
